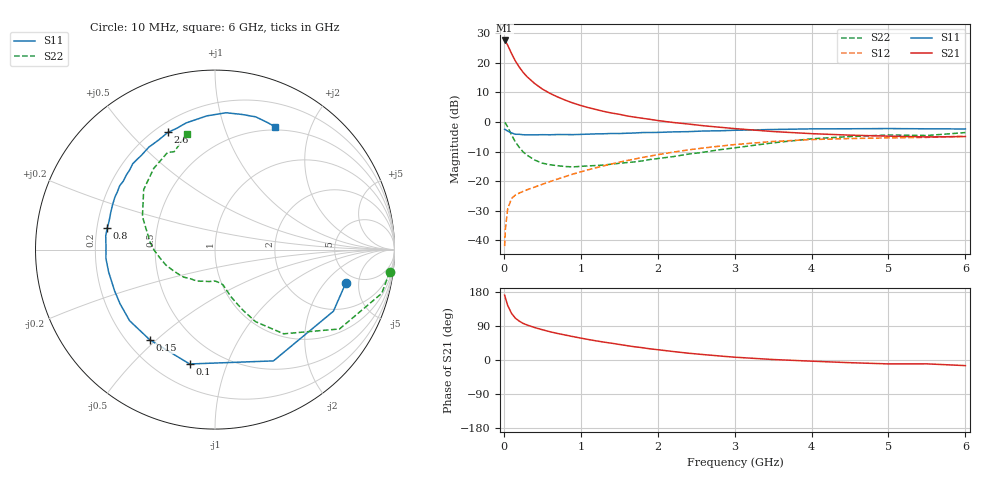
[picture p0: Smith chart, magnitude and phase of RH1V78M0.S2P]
! SIEMENS Small Signal Semiconductors
! BFR106
! Si NPN RF Bipolar Junction Transistor in SOT23
! VCE = 1.75 V  IC = 8 mA
! Common Emitter S-Parameters:  August  1996
# GHz  S  MA  R  50
!  f  S11  S21  S12  S22
! GHz  MAG  ANG  MAG  ANG  MAG  ANG  MAG  ANG
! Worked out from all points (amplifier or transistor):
!   36 points, 10 MHz to 6 GHz, reference 50 ohm
!   highest |S21| = 27.5 dB at 10 MHz (marker M1)
!   |S21| within 3 dB of that: start of sweep to 74.89 MHz
!   unconditionally stable (mu >= 1): 514.9 MHz to 2.392 GHz; 4.406 GHz to end of sweep
!   at 250 MHz: K = 0.65, MSG = 20.1 dB, |S12| = -23.4 dB
!   at 1.4 GHz: K = 1.12, MAG = 6.5 dB, |S12| = -14.2 dB
!   at 6 GHz: K = 1.02, MAG = -1.0 dB, |S12| = -4.8 dB
!   S11 on the Smith chart (normalised r, x): 10 MHz: 4.07, -3.44; 100 MHz: 0.34, -0.75; 150 MHz: 0.29, -0.48; 800 MHz: 0.24, +0.09; 2.6 GHz: 0.25, +0.65; 6 GHz: 0.46, +1.50
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0.01  0.7526 -14.1  23.77 171.2  0.008 85.5  0.9813 -7.3
0.02  0.7437 -27.5  23.18 164.1  0.0155 77.3  0.9606 -14.7
0.05  0.7004 -62.3  19.73 143.9  0.0341 62.0  0.8228 -32.5
0.1  0.6527 -102.5  14.33 123.1  0.0511 47.9  0.6053 -50.8
0.15  0.6202 -125.9  10.7 110.3  0.0583 41.7  0.4599 -60.7
0.2  0.6192 -140.2  8.456 102.7  0.063 40.5  0.3737 -65.1
0.25  0.6091 -150.3  6.898 96.7  0.0673 40.6  0.3125 -68.7
0.3  0.6048 -157.7  5.837 92.5  0.0714 42.2  0.2765 -71.3
0.4  0.6056 -168.1  4.467 85.7  0.0796 44.8  0.2279 -74.7
0.5  0.6098 -175.4  3.6 79.9  0.0886 47.9  0.2016 -77.2
0.6  0.6077 178.2  3.038 74.6  0.0985 50.3  0.1897 -80.4
0.8  0.6124 168.7  2.327 65.8  0.1201 53.8  0.1767 -88.5
0.9  0.611 164.8  2.087 61.7  0.132 55.1  0.1745 -91.8
1.1  0.623 156.3  1.744 54.0  0.1561 56.3  0.1813 -101.0
1.3  0.6318 149.4  1.507 47.2  0.1822 56.3  0.1872 -110.2
1.6  0.6454 139.9  1.265 37.9  0.2234 55.0  0.2064 -124.8
2.2  0.6796 122.8  0.98 22.4  0.3092 48.8  0.2599 -152.9
2.6  0.704 111.9  0.862 14.2  0.3642 42.8  0.3088 -170.9
3.5  0.7464 93.5  0.689 1.3  0.4685 27.7  0.4443 155.5
4.5  0.7677 78.9  0.599 -7.1  0.5252 11.1  0.5669 127.0
5.5  0.7661 67.6  0.559 -10.2  0.5488 1.0  0.591 112.7
6  0.7618 63.9  0.567 -14.8  0.5735 -6.2  0.6621 103.5
